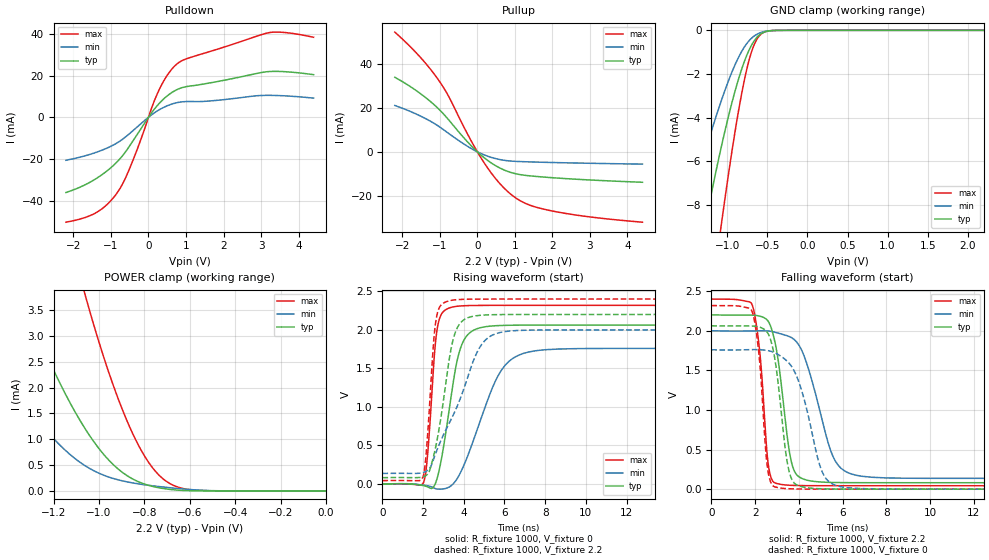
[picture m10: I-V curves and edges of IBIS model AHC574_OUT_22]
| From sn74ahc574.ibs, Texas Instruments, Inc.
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[Model]   AHC574_OUT_22
Model_type  3-state
Enable   Active-Low
Vref =   0
Rref =   1000
Cref =   50p
Vmeas =   1.1
| variable   typ   min   max
C_comp   2.14pF   1.85pF   2.30pF
| C_pullup   3.14pF   1.95pF   3.87pF
| C_pulldown   2.95pF   2.16pF   3.95pF
| C_tri-state   2.14pF   1.85pF   2.30pF
[Temperature Range]   40   100   -40
| Ambient temperature   25   85   -40
[Voltage range]   2.2   2   2.4
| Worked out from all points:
|   slope of the pulldown table from 0 to 0.33 V, typ, clamps not added: 44 ohm
|   slope of the pullup table from 0 to 0.33 V, typ, clamps not added: 72.2 ohm
|   GND clamp passes 1 mA (typ) near -0.74 V on its own axis
|   POWER clamp passes 1 mA (typ) near -1.03 V on its own axis
|   rising waveform, R_fixture 1000, V_fixture 0: 20-80 % time 757ps typ, 1.52ns min, 370ps max; typ from 0 V to 2.06 V
|   falling waveform, R_fixture 1000, V_fixture 2.2: 20-80 % time 583ps typ, 1.12ns min, 396ps max; typ from 2.2 V to 0.081 V
|   rising waveform, R_fixture 1000, V_fixture 2.2: 20-80 % time 753ps typ, 1.73ns min, 357ps max; typ from 0.081 V to 2.2 V
|   falling waveform, R_fixture 1000, V_fixture 0: 20-80 % time 529ps typ, 978ps min, 379ps max; typ from 2.06 V to 0 V
[GND Clamp]
| AHC574_OUT_22
|   Voltage   I(typ)   I(min)   I(max)
-2.2V     -30.11mA   -19.43mA   -44.12mA
-1.52V    -13.84mA   -8.791mA   -21.91mA
-1.29V    -9.159mA   -5.73mA    -14.93mA
-1.265V   -8.684mA   -5.418mA   -14.2mA
-1.085V   -5.493mA   -3.325mA   -9.156mA
-1.065V   -5.166mA   -3.111mA   -8.623mA
-925mV    -3.065mA   -1.755mA   -5.123mA
-815mV    -1.711mA   -928.2uA   -2.779mA
-715mV    -799.4uA   -422.3uA   -1.186mA
-630mV    -317.6uA   -179uA     -403.3uA
-420mV    -9.481uA   -7.045uA   -6.132uA
2.2V      3.397nA    2.027nA    6.047nA
[POWER Clamp]
| AHC574_OUT_22
|   Voltage   I(typ)   I(min)   I(max)
-2.2V     17.29mA    9.959mA    32.8mA
-1.615V   7.306mA    3.841mA    15.64mA
-1.345V   3.836mA    1.825mA    9.176mA
-1.195V   2.295mA    991.6uA    6.126mA
-1.07V    1.269mA    513.9uA    3.942mA
-1.055V   1.164mA    471.6uA    3.705mA
-955mV    589.1uA    266uA      2.273mA
-865mV    265.4uA    165.8uA    1.242mA
-795mV    126.3uA    116.9uA    645.9uA
-715mV    45.51uA    74.62uA    224.9uA
-570mV    2.157uA    18.48uA    12.08uA
-24.94fV  3.397nA    1.192nA    9.66nA
[Pulldown]
| AHC574_OUT_22
|   Voltage   I(typ)   I(min)   I(max)
-2.2V     -36.15mA   -20.65mA   -50.41mA
-1.39V    -29.41mA   -16.83mA   -45.78mA
-1.1V     -25.7mA    -14.77mA   -41.85mA
-835mV    -21.4mA    -12.31mA   -36.31mA
-660mV    -17.76mA   -10.13mA   -30.96mA
-460mV    -12.63mA   -7.159mA   -22.77mA
275mV     6.439mA    3.482mA    12.85mA
530mV     10.71mA    5.735mA    20.96mA
785mV     13.5mA     7.111mA    25.98mA
3.2V      21.96mA    10.54mA    40.62mA
3.665V    21.88mA    10.27mA    40.67mA
4.4V      20.47mA    9.205mA    38.44mA
[Pullup]
| AHC574_OUT_22
|   Voltage   I(typ)   I(min)   I(max)
-2.2V     33.76mA    20.98mA    54.23mA
-1.57V    27.02mA    16.64mA    43.76mA
-1.085V   20.28mA    12.16mA    33.71mA
-790mV    14.98mA    8.639mA    25.89mA
-230mV    3.927mA    2.157mA    7.028mA
155mV     -2.31mA    -1.192mA   -4.298mA
550mV     -6.885mA   -3.325mA   -13.44mA
945mV     -9.603mA   -4.245mA   -19.92mA
1.36V     -10.81mA   -4.542mA   -23.91mA
1.985V    -11.71mA   -4.832mA   -26.76mA
3.005V    -12.76mA   -5.193mA   -29.5mA
4.4V      -13.79mA   -5.571mA   -31.87mA
[Ramp]
| AHC574_OUT_22
| variable   typ   min   max
dV/dt_r   1.27/7.81E-10   1.10/1.57E-09   1.40/3.79E-10
dV/dt_f   1.27/5.85E-10   1.12/1.12E-09   1.41/3.98E-10
R_load = 1000
[Rising Waveform]
| AHC574_OUT_22
R_fixture =   1000
C_fixture =   0
L_fixture =   0
V_fixture =   0
V_fixture_min = 0
V_fixture_max = 0
|   Time   V(typ)   V(min)   V(max)
0s        692.6pV    1.245nV    346.6pV
2.015ns   -21.53mV   -15.28mV   14.57mV
2.195ns   -35.34mV   -22.38mV   308mV
2.555ns   -21.03mV   -55.14mV   1.675V
2.705ns   88.41mV    -66.23mV   2.033V
3.53ns    1.401V     16.55mV    2.301V
4.19ns    1.936V     363.8mV    2.315V
5.78ns    2.057V     1.448V     2.318V
7.52ns    2.062V     1.729V     2.318V
50ns      2.063V     1.76V      2.318V
[Falling Waveform]
| AHC574_OUT_22
R_fixture =   1000
C_fixture =   0
L_fixture =   0
V_fixture =   2.2
V_fixture_min = 2
V_fixture_max = 2.4
|   Time   V(typ)   V(min)   V(max)
0s        2.2V       2V         2.4V
1.875ns   2.197V     1.997V     2.32V
2.21ns    2.184V     1.999V     1.744V
2.625ns   2.108V     1.996V     271.1mV
3.195ns   1.328V     1.959V     59.95mV
3.57ns    469.8mV    1.926V     49.58mV
3.895ns   183.9mV    1.859V     46.39mV
5.595ns   84.4mV     393.2mV    43.53mV
6.875ns   81.66mV    163.2mV    43.43mV
50ns      81.34mV    135.9mV    43.42mV
[Rising Waveform]
| AHC574_OUT_22
R_fixture =   1000
C_fixture =   0
L_fixture =   0
V_fixture =   2.2
V_fixture_min = 2
V_fixture_max = 2.4
|   Time   V(typ)   V(min)   V(max)
0s        81.34mV    135.9mV    43.42mV
2.01ns    93.36mV    149.2mV    103.5mV
2.17ns    115.2mV    167.9mV    457.1mV
2.5ns     345.6mV    308.8mV    1.786V
2.63ns    495.2mV    405.7mV    2.121V
3.4ns     1.788V     851.2mV    2.384V
3.87ns    2.101V     1.139V     2.395V
4.835ns   2.19V      1.794V     2.4V
6.26ns    2.199V     1.985V     2.4V
50ns      2.2V       2V         2.4V
[Falling Waveform]
| AHC574_OUT_22
R_fixture =   1000
C_fixture =   0
L_fixture =   0
V_fixture =   0
V_fixture_min = 0
V_fixture_max = 0
|   Time   V(typ)   V(min)   V(max)
0s        2.063V     1.76V      2.318V
1.87ns    2.06V      1.762V     2.238V
2.185ns   2.047V     1.761V     1.677V
2.585ns   1.968V     1.749V     235mV
3.125ns   1.163V     1.688V     16.42mV
3.45ns    372mV      1.619V     6.79mV
3.735ns   96.45mV    1.519V     3.494mV
5.075ns   4.526mV    214.5mV    252.8uV
6.12ns    672uV      22.08mV    37.66uV
50ns      3.573nV    22.73nV    -47.42pV
